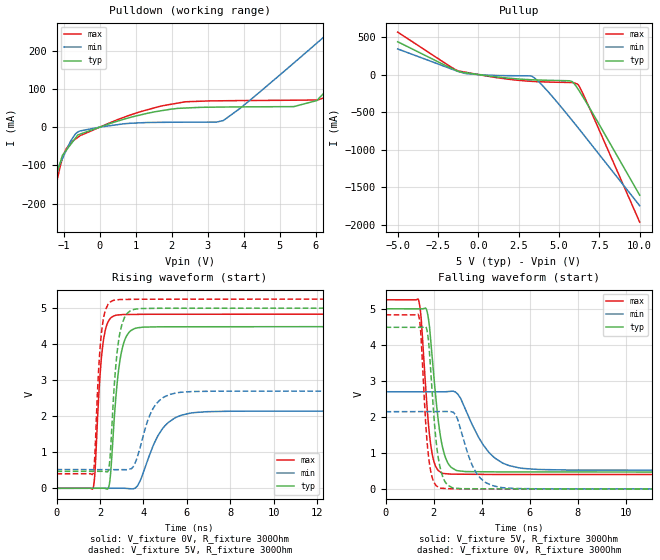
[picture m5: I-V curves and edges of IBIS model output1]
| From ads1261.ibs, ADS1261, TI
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|   output1 Model
[Model]   output1
Model_type   Output
Polarity   Non-Inverting
Vmeas = 2.5
Vref = 0
Cref = 20pF
Rref = 100000
|   typ   min   max
C_comp   3.088pF   2.777pF   3.324pF
|  Where Nom  PVT is Nominal Process,   5V,  27C
|   Fast PVT is Strong Process,   5.25V, -40C
|   Slow PVT is Weak Process,   2.7V, 135C
[Voltage Range]   5   2.7   5.25
|Junction Temperature
[Temperature Range]   27   135   -40
[Pullup Reference]   5   2.7   5.25
[Pulldown Reference]   0   0   0
[Power Clamp Reference]   5   2.7   5.25
[GND Clamp Reference]   0   0   0
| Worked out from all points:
|   slope of the pulldown table from 0 to 0.75 V, typ, clamps not added: 32.8 ohm
|   slope of the pullup table from 0 to 0.75 V, typ, clamps not added: 35 ohm
|   falling waveform, V_fixture 5V, R_fixture 300Ohm: 20-80 % time 424ps typ, 1.1ns min, 325ps max; typ from 5 V to 0.47 V
|   rising waveform, V_fixture 0V, R_fixture 300Ohm: 20-80 % time 385ps typ, 978ps min, 295ps max; typ from 0 V to 4.49 V
|   rising waveform, V_fixture 5V, R_fixture 300Ohm: 20-80 % time 340ps typ, 733ps min, 265ps max; typ from 0.47 V to 5 V
|   falling waveform, V_fixture 0V, R_fixture 300Ohm: 20-80 % time 339ps typ, 699ps min, 272ps max; typ from 4.49 V to 0 V
[Pulldown]
|   Voltage   I(typ)   I(min)   I(max)
-5V       -1.52A     -1.098A    -1.984A
-2.162V   -463.2mA   -346mA     -601.1mA
-1.678V   -287.6mA   -225.6mA   -371.2mA
-1.25V    -139.9mA   -124.4mA   -167.5mA
-1.036V   -73.59mA   -81.88mA   -81.04mA
-607.2mV  -20.35mA   -12.37mA   -26.7mA
1.643V    41.8mA     12.44mA    53.6mA
3.438V    52.55mA    17.33mA    68.94mA
6.035V    69.51mA    219.6mA    71mA
6.892V    161mA      290.8mA    162mA
8.096V    293mA      391.5mA    337.5mA
10V       524.4mA    558.4mA    641mA
[Pullup]
|   Voltage   I(typ)   I(min)   I(max)
-5V       436.6mA    340.9mA    564.9mA
-1.25V    42.38mA    40.94mA    48.92mA
92.87mV   -2.779mA   -1.339mA   -3.569mA
3.33V     -69.54mA   -23.91mA   -90.53mA
4.292V    -76.26mA   -219.9mA   -99.32mA
5.696V    -84.69mA   -579.2mA   -105.6mA
5.915V    -114.6mA   -637.1mA   -110.3mA
6.126V    -176.7mA   -693.2mA   -124.5mA
6.25V     -216.5mA   -726.4mA   -155.1mA
6.501V    -304.1mA   -794.6mA   -262.7mA
7.006V    -485.7mA   -931.7mA   -502.2mA
10V       -1.605A    -1.745A    -1.964A
[Ramp]
R_load = 300
|   typ   min   max
dV/dt_r   2.69214/3.8448e-10   1.2879/9.74421e-10   2.89953/2.94369e-10
dV/dt_f   2.7178/4.22619e-10   1.30746/1.09876e-09   2.90858/3.23632e-10
[Falling Waveform]
V_fixture = 5V
V_fixture_min = 2.7V
V_fixture_max = 5.25V
R_fixture = 300Ohm
C_fixture = 0F
|   Time   V(typ)   V(min)   V(max)
0s        5V         2.7V       5.25V
1.38ns    4.999V     2.699V     5.228V
1.485ns   4.999V     2.699V     4.694V
1.693ns   4.999V     2.699V     2.588V
1.869ns   4.188V     2.699V     1.273V
2.336ns   1.267V     2.699V     448mV
2.92ns    525.6mV    2.684V     415.8mV
4.27ns    481.1mV    1.041V     408.6mV
5.535ns   477.9mV    592.7mV    407.2mV
20ns      470.3mV    520.7mV    402.4mV
[Rising Waveform]
V_fixture = 0V
V_fixture_min = 0V
V_fixture_max = 0V
R_fixture = 300Ohm
C_fixture = 0F
|   Time   V(typ)   V(min)   V(max)
0s        54.22uV    419uV      5.495uV
1.685ns   1.255mV    858.2uV    703.2uV
2.128ns   1.571mV    973.7uV    3.954V
2.432ns   104.3mV    1.053mV    4.673V
2.662ns   1.96V      1.113mV    4.787V
3.054ns   3.944V     1.215mV    4.82V
3.655ns   4.442V     22.3mV     4.825V
4.846ns   4.481V     1.623V     4.828V
6.135ns   4.481V     2.082V     4.829V
20ns      4.487V     2.147V     4.833V
[Rising Waveform]
V_fixture = 5V
V_fixture_min = 2.7V
V_fixture_max = 5.25V
R_fixture = 300Ohm
C_fixture = 0F
|   Time   V(typ)   V(min)   V(max)
0s        470.3mV    520.7mV    402.4mV
1.685ns   471.4mV    518.3mV    410.3mV
2.062ns   471.7mV    517.8mV    4.262V
2.399ns   518.4mV    517.3mV    5.123V
2.554ns   1.751V     517.1mV    5.198V
2.92ns    4.31V      516.5mV    5.237V
3.512ns   4.952V     582.9mV    5.242V
4.446ns   4.992V     2.211V     5.245V
5.535ns   4.995V     2.648V     5.246V
20ns      5V         2.7V       5.25V
[Falling Waveform]
|Gnd
V_fixture = 0V
V_fixture_min = 0V
V_fixture_max = 0V
R_fixture = 300Ohm
C_fixture = 0F
|   Time   V(typ)   V(min)   V(max)
0s        4.487V     2.147V     4.833V
1.37ns    4.486V     2.15V      4.827V
1.46ns    4.486V     2.15V      4.377V
1.798ns   4.023V     2.151V     842.8mV
2.052ns   1.674V     2.151V     150mV
2.244ns   676.6mV    2.152V     36.47mV
2.764ns   43.5mV     2.141V     12.38mV
3.759ns   11.28mV    464.3mV    8.382mV
4.718ns   7.338mV    55.31mV    4.525mV
20ns      54.25uV    419.1uV    5.518uV
